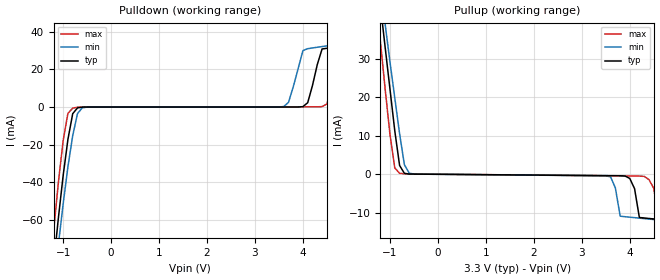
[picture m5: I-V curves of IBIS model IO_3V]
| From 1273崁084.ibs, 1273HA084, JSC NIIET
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[Model]   IO_3V
Model_type I/O
Polarity   Non-Inverting
Vinl =   0.80V
Vinh =   2.10V
C_comp   1.984800pF   1.899400pF   2.077500pF
[Temperature Range]   25   -60   85
[Voltage Range]   3.30V   3.00V   3.60V
[Pullup Reference]   3.30V   3.00V   3.60V
[Pulldown Reference]   0.00V   0.00V   0.00V
[POWER Clamp Reference]   3.30V   3.00V   3.60V
[GND Clamp Reference]   0.00V   0.00V   0.00V
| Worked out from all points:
|   slope of the pullup table from 0 to 0.495 V, typ, clamps not added: 10.1 kohm
[Pullup]
| Voltage   I(typ)   I(min)   I(max)
-3.6V     465.9mA    414.5mA    536.2mA
-1.3V     55.65mA    61.19mA    46.98mA
-1.2V     43.92mA    49.53mA    34.48mA
-1.1V     32.9mA     38.91mA    22.06mA
-900mV    11.28mA    19.85mA    1.659mA
-800mV    2.301mA    10.57mA    261.1uA
-600mV    65.76uA    305.8uA    99.39uA
3.5V      -348.4uA   -385.5uA   -380.2uA
3.9V      -434uA     -11.02mA   -428.4uA
4.3V      -11.35mA   -11.52mA   -535.2uA
4.6V      -11.73mA   -11.88mA   -11.35mA
7.2V      -15.16mA   -15.16mA   -14.57mA
[Pulldown]
| Voltage   I(typ)   I(min)   I(max)
-3.6V     -895.1mA   -825.2mA   -997.8mA
-1.2V     -84.12mA   -96.75mA   -66.66mA
-1.1V     -59.42mA   -73.61mA   -40.48mA
-1V       -36.65mA   -51.78mA   -18mA
-800mV    -3.542mA   -15.23mA   -615.6uA
-700mV    -476.8uA   -3.475mA   -65.98uA
-500mV    -5.225uA   -41.23uA   -9.554uA
3.6V      2.574uA    256.9uA    76.9uA
4V        204uA      30.03mA    86.62uA
4.4V      30.91mA    32.2mA     220.6uA
4.8V      32.37mA    33.67mA    27.29mA
7.2V      41.34mA    42.28mA    34.59mA
[Ramp]
| variable   typ   min   max
dV/dt_r   1.1447/1.0797n   0.8477/2.2066n   1.3962/0.5592n
dV/dt_f   1.1301/1.6088n   0.6820/2.6083n   1.4669/0.8614n
R_load = 1500ohms
